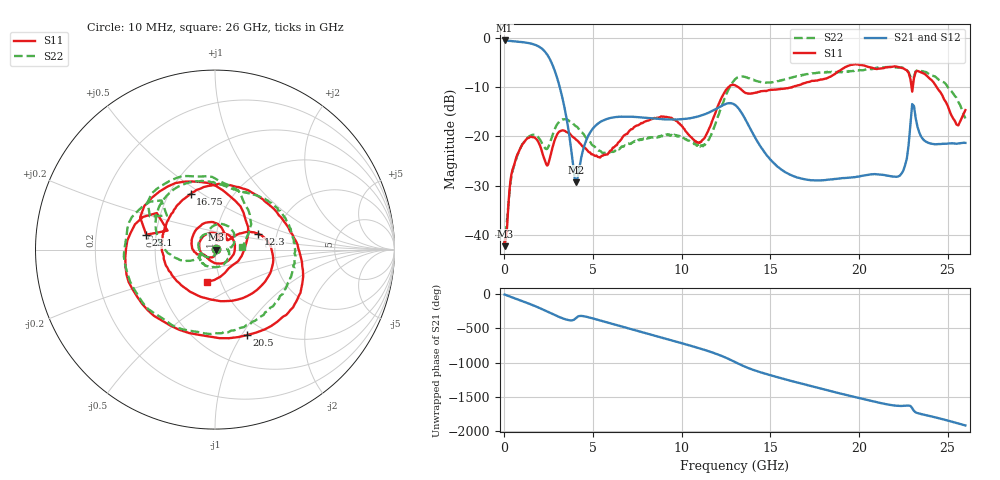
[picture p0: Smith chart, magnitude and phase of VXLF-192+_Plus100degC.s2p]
! Mini-Circuits
! S2P DATA File Format
! Type: LOW PASS FILTER
! Model: VXLF-192+
! All S Parameters are in dB deg format
! TEST CONDITIONS: INPUT POWER = 0 dBm @ Temperature = +100deg C
# MHz S dB R 50
!Frequency  S11 dB  S11 DEG  S21 dB  S21 DEG  S12 dB  S12 DEG  S22 dB  S22 DEG
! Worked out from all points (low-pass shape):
!   1260 points, 10 MHz to 26 GHz, reference 50 ohm
!   highest |S21| = -0.51 dB at 10 MHz (marker M1); lowest = -29.3 dB at 4.04 GHz (marker M2)
!   |S21| within 3 dB of the highest: start of sweep to 2.434 GHz
!   lowest |S11| = -42.3 dB at 30 MHz (marker M3), VSWR 1.02, Z = 50.8 - j0.0298 ohm
!   |S11| at or under -10 dB: start of sweep to 12.64 GHz; 13.19 GHz to 16.23 GHz (3.039 GHz wide, 20.7 % of centre); 24.38 GHz to end of sweep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
!   |S22| runs from -41.7 to -5.9 dB; largest |S21 - S12| = 0.0029
!   S11 on the Smith chart (normalised r, x): 10 MHz: 1.02, +0.00; 12.3 GHz: 1.60, +0.30; 16.75 GHz: 0.64, +0.45; 20.5 GHz: 0.82, -1.06; 23.1 GHz: 0.44, +0.09; 26 GHz: 0.86, -0.32
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10  -41.51 13.1  -0.51 -1.0  -0.51 -1.0  -41.69 11.0
30  -42.33 -2.2  -0.51 -3.0  -0.51 -3.0  -41.61 -1.6
380  -28.04 -100.4  -0.63 -36.6  -0.63 -36.5  -28.48 -104.9
890  -22.45 -160.0  -0.80 -85.5  -0.80 -85.5  -22.45 -159.2
1700  -20.25 106.2  -1.35 -167.8  -1.35 -167.8  -19.62 130.5
2410  -25.93 73.5  -3.38 109.7  -3.38 109.7  -22.54 108.4
2960  -19.70 59.1  -7.98 43.3  -7.98 43.3  -17.69 95.3
4040  -20.70 -48.0  -29.34 15.8  -29.34 15.8  -17.98 28.7
4350  -21.82 -72.8  -24.04 44.7  -24.04 44.7  -19.21 16.9
8680  -16.21 122.8  -16.45 98.5  -16.44 98.6  -20.07 -97.2
11000  -21.35 38.7  -15.88 -71.8  -15.86 -71.9  -21.76 -165.5
12300  -11.78 20.0  -13.71 171.8  -13.69 171.3  -13.44 -165.9
13050  -9.70 -38.1  -13.74 81.3  -13.84 80.8  -8.29 146.2
14400  -10.94 -159.6  -21.81 -59.8  -21.88 -59.0  -8.90 81.0
16750  -9.43 113.8  -28.59 128.8  -28.52 129.3  -7.67 32.1
17350  -8.71 86.5  -28.92 88.6  -28.88 88.9  -7.17 15.3
19150  -6.11 -10.8  -28.48 -29.0  -28.49 -29.1  -6.87 -53.2
20500  -5.87 -69.4  -27.86 -112.4  -27.87 -111.9  -6.30 -116.2
21700  -5.91 -143.5  -28.03 179.3  -27.98 179.5  -5.91 -168.1
23100  -8.14 167.8  -13.86 87.9  -13.82 88.1  -7.80 153.0
24700  -11.69 52.4  -21.53 -32.3  -21.53 -32.3  -8.92 72.4
26000  -14.66 -103.8  -21.33 -125.2  -21.39 -125.0  -16.37 5.3
